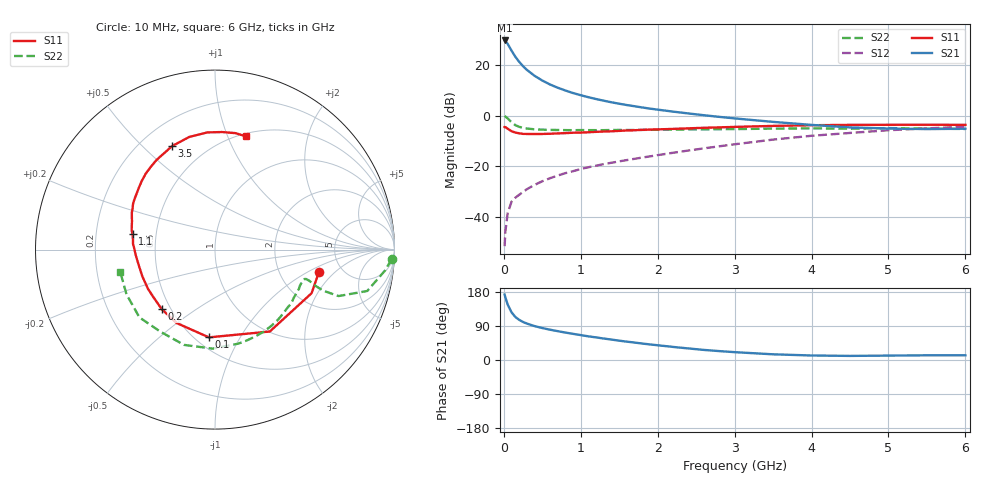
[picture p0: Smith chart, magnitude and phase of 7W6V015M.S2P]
! Infineon Technologies  Discrete & RF Semiconductors
! BFS17W
! Si NPN RF Bipolar Junction Transistor in SOT323
! VCE = 6 V  IC = 15 mA
! Common Emitter S-Parameters:  August  1999
# GHz  S  MA  R  50
!  f  S11  S21  S12  S22
! GHz  MAG  ANG  MAG  ANG  MAG  ANG  MAG  ANG
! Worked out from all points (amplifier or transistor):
!   36 points, 10 MHz to 6 GHz, reference 50 ohm
!   highest |S21| = 29.7 dB at 10 MHz (marker M1)
!   |S21| within 3 dB of that: start of sweep to 80.75 MHz
!   unconditionally stable (mu >= 1): 351.1 MHz to 2.164 GHz; 5.338 GHz to end of sweep
!   at 250 MHz: K = 0.90, MSG = 24.9 dB, |S12| = -30.2 dB
!   at 1.4 GHz: K = 1.16, MAG = 9.5 dB, |S12| = -18.7 dB
!   at 6 GHz: K = 1.04, MAG = -1.6 dB, |S12| = -4.4 dB
!   S11 on the Smith chart (normalised r, x): 10 MHz: 3.37, -1.29; 100 MHz: 0.58, -0.75; 200 MHz: 0.45, -0.37; 1.1 GHz: 0.37, +0.08; 3.5 GHz: 0.33, +0.62; 6 GHz: 0.53, +1.17
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0.01  0.5925 -12.1  30.67 172.7  0.0026 79.6  0.9856 -3.1
0.02  0.5905 -24.3  30.01 165.2  0.0051 81.6  0.9547 -7.0
0.05  0.5491 -56.2  26.24 146.3  0.0117 68.0  0.8792 -15.2
0.1  0.4902 -94.0  19.29 125.8  0.0198 61.0  0.7355 -20.6
0.15  0.4616 -117.5  14.57 113.5  0.0237 58.2  0.6452 -20.8
0.2  0.4452 -131.7  11.55 105.9  0.0271 58.4  0.5988 -19.9
0.25  0.4337 -142.1  9.471 100.3  0.0308 59.2  0.5697 -18.9
0.3  0.4327 -149.5  8.012 96.1  0.0349 60.8  0.5542 -18.3
0.4  0.4315 -159.8  6.116 89.4  0.0425 63.8  0.5338 -17.9
0.5  0.4325 -166.9  4.936 84.3  0.0501 65.4  0.5264 -18.1
0.6  0.4368 -171.9  4.123 80.0  0.0575 67.2  0.5209 -18.9
0.7  0.4436 -176.5  3.562 76.1  0.065 68.3  0.518 -20.2
0.9  0.4577 176.1  2.792 69.0  0.0793 69.3  0.514 -23.3
1.1  0.4676 169.4  2.307 62.4  0.0949 70.3  0.5149 -27.2
1.3  0.4832 163.6  1.968 56.6  0.1096 70.6  0.5144 -31.6
1.6  0.5076 155.9  1.614 48.4  0.1317 71.6  0.5176 -38.4
2.2  0.5446 141.6  1.197 34.5  0.1836 72.7  0.5285 -54.0
2.8  0.5839 127.7  0.943 23.5  0.2464 71.0  0.5365 -70.8
3.5  0.6243 112.5  0.75 15.0  0.3345 66.0  0.5519 -91.3
4.5  0.6543 93.8  0.583 10.8  0.4527 53.6  0.5493 -123.5
5.5  0.6587 80.1  0.54 12.4  0.5581 40.5  0.5525 -153.2
6  0.6541 74.7  0.549 12.4  0.5998 34.1  0.5422 -166.4
